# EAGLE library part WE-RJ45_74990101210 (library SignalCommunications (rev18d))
Order Code 74990101210 Design THT xBase-T 10/100 Base-T Ports 1x1 Vertical Application Standard Tab Position Vertical LED (Left-Right) Yellow-Green EMI Fingers No Details see: http://katalog.we-online.de/en/pbs/WE-LAN_RJ45/74990101210? Updated by Yingchun Shan 2016-08-26 2016(C) Würth Elektronik
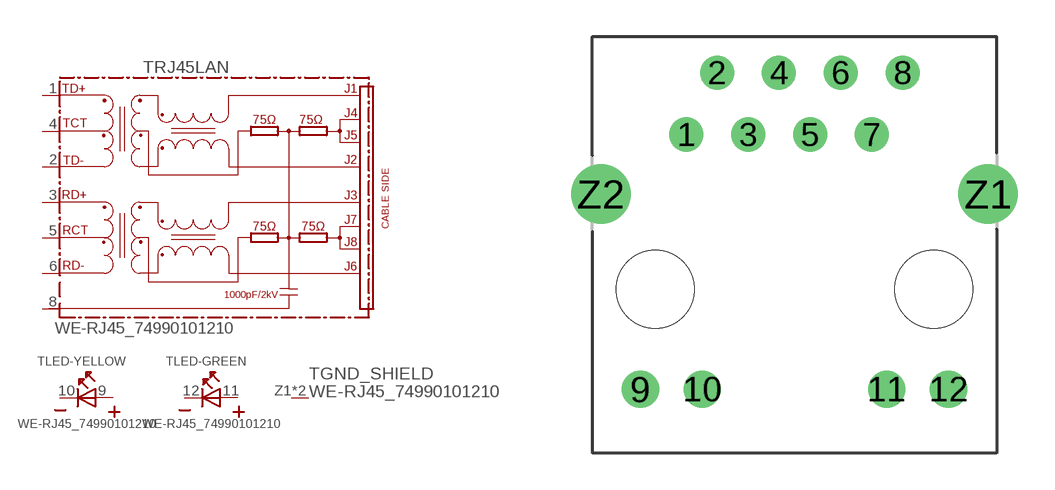
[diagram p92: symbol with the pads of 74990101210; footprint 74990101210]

Designator prefix T; gates RJ45LAN=74990X-THT-10/100-T LED-YELLOW=LED2PIN LED-GREEN=LED2PIN GND_SHIELD=GND_PIN

## WE-RJ45_74990101210 (COMPANY-URL: http://www.we-online.de; CREATED-BY: Christin Zierenner; CREATED-DATE: AUG 2012; DATASHEET-URL: http://katalog.we-online.de/kataloge/eisos/media/pdf/74990101210.pdf; MANUFACTURER: Würth Elektronik eiSos GmbH)  [74990101210]
1  RJ45LAN:TD+
2  RJ45LAN:TD-
3  RJ45LAN:RD+
4  RJ45LAN:TCT
5  RJ45LAN:RCT
6  RJ45LAN:RD-
8  RJ45LAN:8
9  LED-YELLOW:A  pas
10  LED-YELLOW:K  pas
11  LED-GREEN:A  pas
12  LED-GREEN:K  pas
Z1  GND_SHIELD:1  pwr
Z2  GND_SHIELD:1  pwr

## Footprint 74990101210 (pad centres in mm)
MAX HEIGHT=17.50mm VERTICAL MOUNT PORTS----1X1 LED --YES
drill 0.89: 1 -4.44,6.35; 2 -3.18,8.89; 3 -1.9,6.35; 4 -0.64,8.89; 5 0.64,6.35; 6 1.9,8.89; 7 3.18,6.35; 8 4.44,8.89
drill 1.02: 9 -6.325,-4.11; 10 -3.785,-4.11; 11 3.785,-4.11; 12 6.325,-4.11
drill 1.63: Z1 7.95,3.9; Z2 -7.95,3.9
hole 3.2 at -5.715,0
hole 3.2 at 5.715,0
